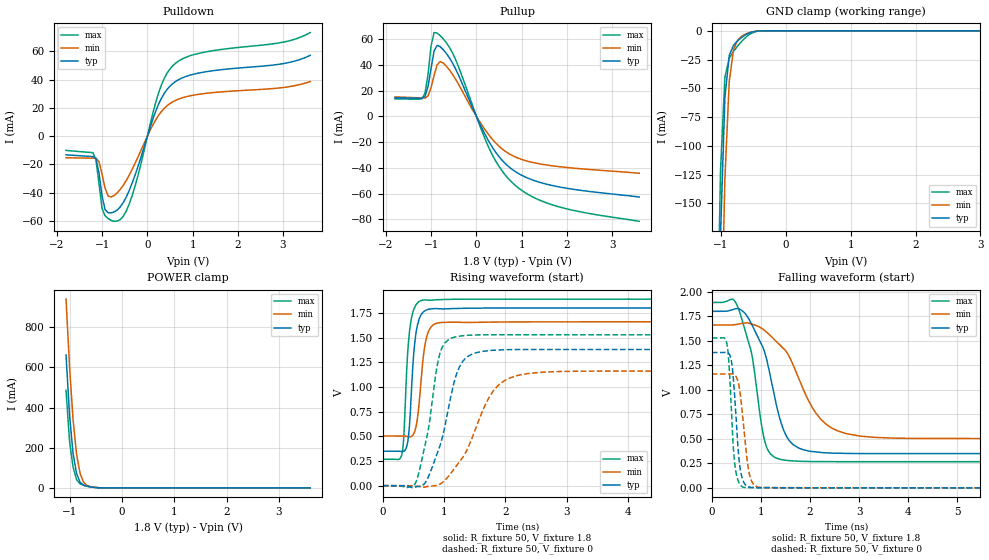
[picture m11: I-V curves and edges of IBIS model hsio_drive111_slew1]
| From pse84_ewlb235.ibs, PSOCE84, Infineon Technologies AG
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[Model] hsio_drive111_slew1
Model_type I/O
Enable   Active-High
Vinl  =  0.54
Vinh  =  1.26
Vmeas =  0.9
Cref  =  15pF
| Capacitance   typ   min   max
C_comp   1.183861e-12   1.145095e-12   1.230403e-12
| Variables   typ   min   max
[GND Clamp Reference]   0   0   0
[POWER Clamp Reference]   1.8   1.66   1.89
[Pulldown Reference]   0   0   0
[Pullup Reference]   1.8   1.66   1.89
[Temperature Range]   25   125   -40
[Voltage Range]   1.8   1.66   1.89
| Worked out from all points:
|   slope of the pulldown table from 0 to 0.27 V, typ, clamps not added: 11.2 ohm
|   slope of the pullup table from 0 to 0.27 V, typ, clamps not added: 14.1 ohm
|   GND clamp passes 1 mA (typ) near -0.51 V on its own axis
|   POWER clamp passes 1 mA (typ) near -0.47 V on its own axis
|   falling waveform, R_fixture 50, V_fixture 1.8: 20-80 % time 462ps typ, 718ps min, 330ps max; typ from 1.8 V to 0.349 V
|   falling waveform, R_fixture 50, V_fixture 0: 20-80 % time 116ps typ, 146ps min, 100ps max; typ from 1.38 V to 0 V
|   rising waveform, R_fixture 50, V_fixture 1.8: 20-80 % time 94.3ps typ, 112ps min, 85.9ps max; typ from 0.349 V to 1.8 V
|   rising waveform, R_fixture 50, V_fixture 0: 20-80 % time 332ps typ, 529ps min, 238ps max; typ from 0 V to 1.38 V
[GND Clamp]
| Voltage   I(typ)   I(min)   I(max)
-1.137V   -688mA     -831.1mA   -596.4mA
-1.07V    -398.5mA   -545.5mA   -312.5mA
-1.003V   -176.8mA   -300mA     -120.9mA
-936.6mV  -57.93mA   -128.6mA   -40.51mA
-869.7mV  -21.44mA   -44.12mA   -23.78mA
-802.8mV  -12.54mA   -16.03mA   -17.79mA
-735.9mV  -8.37mA    -7.69mA    -12.93mA
-669mV    -5.28mA    -4.356mA   -8.606mA
-535.2mV  -1.316mA   -1.208mA   -2.332mA
-401.4mV  -73.56uA   -132.2uA   -119.3uA
3.6V      0A         0A         0A
[POWER Clamp]
| Voltage   I(typ)   I(min)   I(max)
-1.07V    662.2mA    940mA      485.7mA
-1.003V   363.7mA    605.6mA    233mA
-936.6mV  172.7mA    341mA      103.9mA
-869.7mV  72.74mA    168.6mA    41.65mA
-802.8mV  28.31mA    73.56mA    19.99mA
-735.9mV  13.11mA    28.55mA    13.36mA
-669mV    7.76mA     11.5mA     8.963mA
-535.2mV  2.357mA    2.863mA    2.668mA
-334.5mV  34.33uA    127.4uA    15.59uA
3.6V      0A         0A         0A
[Pulldown]
| Voltage   I(typ)   I(min)   I(max)
-1.8V     -13.25mA   -15.29mA   -10.11mA
-1.204V   -14.48mA   -15.56mA   -11.72mA
-1.137V   -15.81mA   -15.56mA   -17.11mA
-1.003V   -42.36mA   -26.9mA    -51.24mA
-936.6mV  -52.04mA   -36.88mA   -56.38mA
-869.7mV  -54.22mA   -42.29mA   -58.38mA
-669mV    -52.31mA   -40.21mA   -60.2mA
-401.4mV  -38.39mA   -27.58mA   -48.03mA
248.3mV   22.71mA    14.73mA    30.76mA
558.6mV   37.11mA    24.24mA    49.74mA
1.117V    44.51mA    29.5mA     58.4mA
3.6V      57.13mA    38.61mA    73.29mA
[Pullup]
| Voltage   I(typ)   I(min)   I(max)
-1.8V     14.54mA    15.19mA    13.64mA
-1.204V   14.13mA    14.36mA    13.74mA
-1.137V   15.76mA    14.25mA    18.07mA
-1.07V    23.08mA    16.06mA    32.75mA
-1.003V   37.57mA    22.35mA    54.9mA
-936.6mV  50.85mA    32.04mA    65.25mA
-869.7mV  55.28mA    40.1mA     64.89mA
-468.3mV  37.53mA    29.41mA    44.86mA
310.3mV   -21.62mA   -15.99mA   -26.97mA
806.9mV   -41.6mA    -30.63mA   -51.97mA
1.738V    -54.19mA   -38.68mA   -69.42mA
3.6V      -62.69mA   -44.2mA    -81.58mA
[Ramp]
dV/dt_r   0.827825/0.332306n  0.696273/0.529008n  0.917219/0.237611n
dV/dt_f   0.870357/0.462033n  0.693939/0.717988n  0.973864/0.330131n
R_load = 50
[Falling Waveform]
R_fixture = 50
V_fixture = 1.8
V_fixture_min = 1.66
V_fixture_max = 1.89
| Time   V(typ)   V(min)   V(max)
0s        1.8V       1.66V      1.89V
450ps     1.823V     1.663V     1.913V
742ps     1.732V     1.681V     1.492V
1.104ns   1.333V     1.593V     429.1mV
1.37ns    729.7mV    1.464V     294.6mV
1.582ns   478.7mV    1.333V     276.6mV
2.039ns   370.6mV    824.4mV    268.2mV
2.317ns   357.6mV    652.7mV    267.1mV
3.719ns   349.1mV    506.8mV    266.9mV
50ns      349.4mV    503.4mV    266.9mV
[Falling Waveform]
R_fixture = 50
V_fixture = 0
V_fixture_min = 0
V_fixture_max = 0
| Time   V(typ)   V(min)   V(max)
0s        1.38V      1.16V      1.529V
293.4ps   1.382V     1.16V      1.496V
384.9ps   1.325V     1.163V     929.3mV
432.4ps   1.148V     1.161V     441.4mV
494.6ps   704.4mV    1.132V     149.6mV
581.8ps   178.7mV    942.5mV    27.77mV
704.2ps   22.4mV     347.1mV    2.239mV
804.5ps   4.338mV    73.16mV    2.767mV
1.07ns    2.806mV    1.788mV    1.284mV
50ns      10.16nV    749nV      3.622nV
[Rising Waveform]
R_fixture = 50
V_fixture = 1.8
V_fixture_min = 1.66
V_fixture_max = 1.89
| Time   V(typ)   V(min)   V(max)
0s        349.4mV    503.4mV    266.9mV
309.2ps   345.5mV    503.5mV    313.9mV
341.3ps   348.2mV    503.3mV    489.9mV
387.6ps   392.5mV    499.4mV    1.152V
447.8ps   735.2mV    495.3mV    1.625V
531.6ps   1.505V     572.4mV    1.822V
674.8ps   1.767V     1.376V     1.882V
815.6ps   1.793V     1.627V     1.881V
1.136ns   1.794V     1.656V     1.888V
50ns      1.8V       1.66V      1.89V
[Rising Waveform]
R_fixture = 50
V_fixture = 0
V_fixture_min = 0
V_fixture_max = 0
| Time   V(typ)   V(min)   V(max)
0s        10.17nV    735.9nV    3.626nV
508ps     -18.22mV   -2.598mV   2.376mV
705.5ps   42.84mV    -11.92mV   457.8mV
887.8ps   327.8mV    3.599mV    1.22V
966.2ps   473.9mV    28.59mV    1.399V
1.181ns   1.088V     183.2mV    1.506V
1.381ns   1.305V     372.7mV    1.524V
1.896ns   1.375V     1.024V     1.529V
2.932ns   1.38V      1.158V     1.529V
50ns      1.38V      1.16V      1.529V
